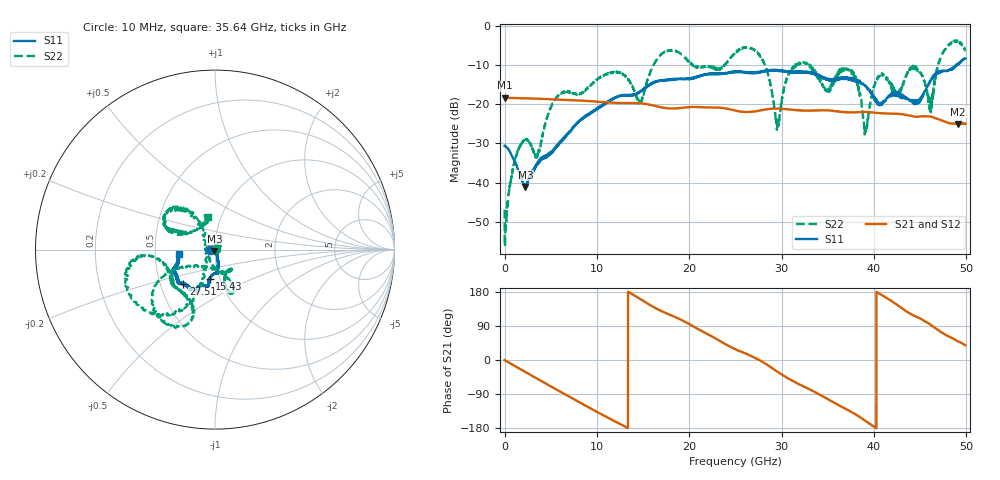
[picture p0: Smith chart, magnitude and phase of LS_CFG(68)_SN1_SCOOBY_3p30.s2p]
!Keysight Technologies,N5245B,MY58422026,A.13.80.08
!Date: Thursday, March 19, 2020 23:48:18
!Correction: S11(Full 2 Port(1,2))
!S21(Full 2 Port(1,2))
!S12(Full 2 Port(1,2))
!S22(Full 2 Port(1,2))
!S2P File: Measurements: S11, S21, S12, S22:
# Hz S DB R 50.0
!freq dBS11 angS11 dBS21 angS21 dBS12 angS12 dBS22 angS22
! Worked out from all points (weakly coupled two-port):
!   4991 points, 10 MHz to 49.91 GHz, reference 50 ohm
!   highest |S21| = -18.28 dB at 10 MHz (marker M1); lowest = -25.0 dB at 49.11 GHz (marker M2)
!   lowest |S11| = -41.1 dB at 2.26 GHz (marker M3), VSWR 1.02, Z = 49.7 - j0.804 ohm
!   |S11| at or under -10 dB: start of sweep to 48.89 GHz; 48.94275 GHz to 48.98731 GHz (44.56 MHz wide, 0.091 % of centre)
!   |S22| runs from -56.3 to -3.6 dB; largest |S21 - S12| = 0.0011
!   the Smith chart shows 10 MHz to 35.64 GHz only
!   S11 on the Smith chart (normalised r, x): 10 MHz: 0.94, -0.01; 15.43 GHz: 0.89, -0.30; 27.51 GHz: 0.66, -0.27; 35.64 GHz: 0.67, -0.03
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1e7  -30.58 -174.8  -18.28 -0.2  -18.27 -0.3  -46.96 12.5
2.26e9  -41.15 -112.5  -18.43 -31.7  -18.42 -31.6  -28.97 35.7
3.51e9  -35.57 -72.8  -18.53 -48.9  -18.52 -48.8  -33.46 145.5
5.51e9  -30.93 -68.0  -18.74 -76.6  -18.73 -76.6  -18.59 -80.2
8.33e9  -23.96 -75.8  -19.03 -114.7  -19.03 -114.6  -17.11 -61.1
1.543e10  -15.56 -100.5  -19.95 150.0  -19.95 150.1  -14.36 -151.7
1.665e10  -14.06 -100.8  -20.58 133.2  -20.57 133.3  -8.00 -147.5
2.496e10  -11.74 -122.3  -21.54 28.8  -21.53 29.0  -6.90 -171.9
2.751e10  -11.67 -132.5  -21.63 1.0  -21.64 1.3  -6.96 -125.3
2.955e10  -11.29 -140.1  -21.08 -30.8  -21.07 -30.5  -25.13 -178.2
3.103e10  -11.61 -145.1  -21.34 -53.0  -21.36 -52.7  -11.03 127.1
3.328e10  -11.92 -156.0  -21.56 -80.7  -21.56 -80.3  -10.72 157.1
3.564e10  -13.92 -174.3  -21.63 -112.1  -21.58 -111.6  -14.47 99.6
3.771e10  -13.82 173.0  -22.03 -139.2  -21.96 -139.3  -12.04 135.7
3.913e10  -15.46 170.5  -21.93 -161.4  -21.91 -161.4  -26.95 -105.1
4.031e10  -19.28 154.9  -22.17 179.5  -22.16 179.3  -13.60 -5.6
4.16e10  -17.82 107.6  -22.33 160.5  -22.36 160.5  -14.26 27.1
4.445e10  -19.35 57.2  -23.15 115.7  -23.16 116.0  -10.42 -14.5
4.615e10  -13.77 10.8  -23.10 92.7  -23.12 92.8  -21.99 -50.3
4.735e10  -11.35 10.1  -24.11 72.4  -24.12 72.6  -7.23 -82.7
4.911e10  -9.70 -12.8  -25.04 49.2  -25.06 49.3  -3.81 -43.9
4.991e10  -8.24 -13.7  -24.93 39.0  -24.95 39.1  -6.11 -28.6
